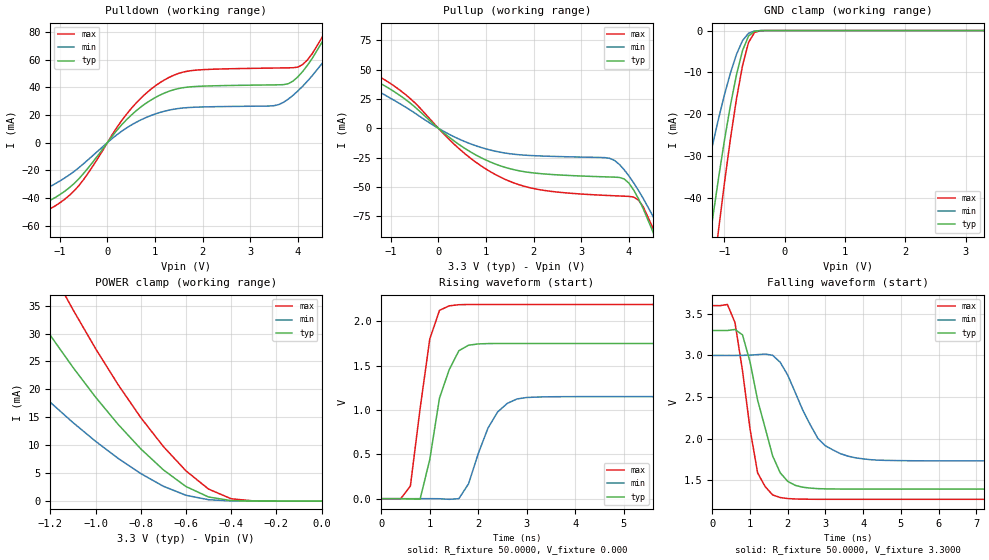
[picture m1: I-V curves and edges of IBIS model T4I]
| IBIS file t4i.ibs created by s2ibis2 version 1.1
| North Carolina State University Electronics Research Laboratory  1995
[IBIS ver]   2.1
[File name]   t4i.ibs
[File Rev]   1.0
[Date]   Wednesday, March 29, 2000
[Source]   From silicon level SPICE at TOSHIBA.
[Notes]   This model does not include the values of Package Model
[Disclaimer]   None.
[Copyright]   Copyright(C) TOSHIBA Corp. 1996-2000. All Rights Reserved
|   Component TC260C
[Component]   TC260C
[Manufacturer]   TOSHIBA
[Package]
| variable   typ   min   max
R_pkg   1.0000f   NA   NA
L_pkg   1.0000fH   NA   NA
C_pkg   1.0000fF   NA   NA
[Pin]  signal_name   model_name   R_pin   L_pin   C_pin
Z   Z   T4I
VDDS   VDDS   POWER
VSS   VSS   GND
| Models and submodels in the file (1): T4I (3-state)
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|   Model T4I
[Model]   T4I
Model_type   3-state
Polarity   Non-Inverting
C_comp   4.2000pF   NA   NA
Vmeas = 1.40V
|Variable   typ   min   max
[Voltage range]  3.3   3.0   3.6
[Temperature Range]   25.0000   100.0000   0.000
[Pullup Reference]   3.3000V   3.0000V   3.6000V
[Pulldown Reference]   0.000V   0.000V   0.000V
[POWER Clamp Reference]   3.3000V   3.0000V   3.6000V
[GND Clamp Reference]   0.000V   0.000V   0.000V
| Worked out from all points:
|   slope of the pulldown table from 0 to 0.495 V, typ, clamps not added: 25.2 ohm
|   slope of the pullup table from 0 to 0.495 V, typ, clamps not added: 31.9 ohm
|   GND clamp passes 1 mA (typ) near -0.57 V on its own axis
|   POWER clamp passes 1 mA (typ) near -0.51 V on its own axis
|   rising waveform, R_fixture 50.0000, V_fixture 0.000: 20-80 % time 408ps typ, 500ps min, 320ps max; typ from 0 V to 1.75 V
|   falling waveform, R_fixture 50.0000, V_fixture 3.3000: 20-80 % time 615ps typ, 821ps min, 454ps max; typ from 3.3 V to 1.39 V
[Pulldown]
| voltage   I(typ)   I(min)   I(max)
-3.3V     -59mA      -58.31mA   -64.86mA
-1.9V     -51.23mA   -43.07mA   -57.58mA
-1V       -37.65mA   -27.81mA   -43.59mA
-500mV    -22.31mA   -15.25mA   -26.74mA
600mV     22.86mA    14.58mA    28.46mA
1.4V      38.26mA    24.15mA    48.77mA
3.6V      41.74mA    27.49mA    53.92mA
3.8V      42.56mA    31.44mA    54.02mA
4.1V      51.34mA    40.69mA    56.35mA
4.7V      84.91mA    66.18mA    89.44mA
5.1V      114.3mA    87.51mA    123mA
6.6V      274.3mA    211.8mA    309.5mA
[Pullup]
| voltage   I(typ)   I(min)   I(max)
-3.3V     71.91mA    86.68mA    73.87mA
-2.1V     55.22mA    51.34mA    59.93mA
-1.1V     35.6mA     27.85mA    40.67mA
-500mV    18.41mA    13.14mA    21.98mA
500mV     -15.68mA   -10.38mA   -19.73mA
1.5V      -34.43mA   -21.67mA   -45.26mA
3.7V      -41.64mA   -27.45mA   -57.55mA
4V        -46.74mA   -40.6mA    -58.07mA
4.2V      -60.02mA   -52.9mA    -61.17mA
4.5V      -87.85mA   -74.56mA   -84.58mA
4.7V      -109.3mA   -90.59mA   -107mA
6.6V      -337.2mA   -276.9mA   -360.7mA
[GND_clamp]
| voltage   I(typ)   I(min)   I(max)
-3.3V     -292.8mA   -217.8mA   -337.5mA
-1.5V     -77.97mA   -49.07mA   -98.95mA
-1.3V     -55.88mA   -34.36mA   -72.74mA
-1.2V     -45.43mA   -27.57mA   -60.12mA
-1.1V     -35.51mA   -21.22mA   -47.98mA
-900mV    -17.87mA   -10.14mA   -25.85mA
-800mV    -10.56mA   -5.698mA   -16.34mA
-700mV    -4.792mA   -2.412mA   -8.394mA
-600mV    -1.302mA   -649uA     -2.833mA
-500mV    -170.7uA   -108.2uA   -443.3uA
-400mV    -13.58uA   -13.64uA   -33.16uA
3.3V      153.9pA    4.45uA     -1.048nA
[POWER_clamp]
| voltage   I(typ)   I(min)   I(max)
-3.3V     189.1mA    135.9mA    229.2mA
-1.7V     62.57mA    39.06mA    82.98mA
-1.6V     55.54mA    34.4mA     74.31mA
-1.3V     35.75mA    21.56mA    49.45mA
-1.2V     29.69mA    17.7mA     41.7mA
-1.1V     23.96mA    14.08mA    34.3mA
-900mV    13.74mA    7.658mA    20.85mA
-800mV    9.367mA    4.936mA    14.97mA
-600mV    2.612mA    1.048mA    5.42mA
-500mV    737.5uA    251.8uA    2.156mA
-400mV    94.87uA    37.87uA    425.3uA
0V        153.9pA    711.8pA    166.4pA
[Ramp]
| variable   typ   min   max
dV/dt_r   1.0489/0.3314n   0.6897/0.4831n   1.3124/0.2690n
dV/dt_f   1.1453/0.5524n   0.7612/0.8651n   1.3990/0.4225n
R_load = 50.0000
[Rising Waveform]
R_fixture = 50.0000
V_fixture = 0.000
V_fixture_min = 0.000
V_fixture_max = 0.000
| time   V(typ)   V(min)   V(max)
0s        0V         0V         0V
600ps     -3.099mV   18.79uV    143.2mV
800ps     -5.757mV   124uV      1.014V
1ns       441.6mV    332.4uV    1.799V
1.2ns     1.132V     -520.1uV   2.121V
1.4ns     1.452V     -7.228mV   2.172V
1.8ns     1.729V     167.6mV    2.187V
2.2ns     1.747V     794.3mV    2.187V
2.8ns     1.748V     1.123V     2.187V
10ns      1.748V     1.149V     2.187V
[Falling Waveform]
R_fixture = 50.0000
V_fixture = 3.3000
V_fixture_min = 3.0000
V_fixture_max = 3.6000
| time   V(typ)   V(min)   V(max)
0s        3.3V       3V         3.6V
400ps     3.3V       3V         3.613V
600ps     3.312V     3V         3.396V
800ps     3.248V     3.001V     2.816V
1.2ns     2.463V     3.01V      1.588V
1.6ns     1.79V      3.002V     1.321V
2.2ns     1.437V     2.553V     1.273V
2.8ns     1.397V     2.002V     1.269V
3.4ns     1.392V     1.818V     1.268V
10ns      1.391V     1.731V     1.268V
